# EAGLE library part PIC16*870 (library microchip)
MICROCONTROLLER flash type
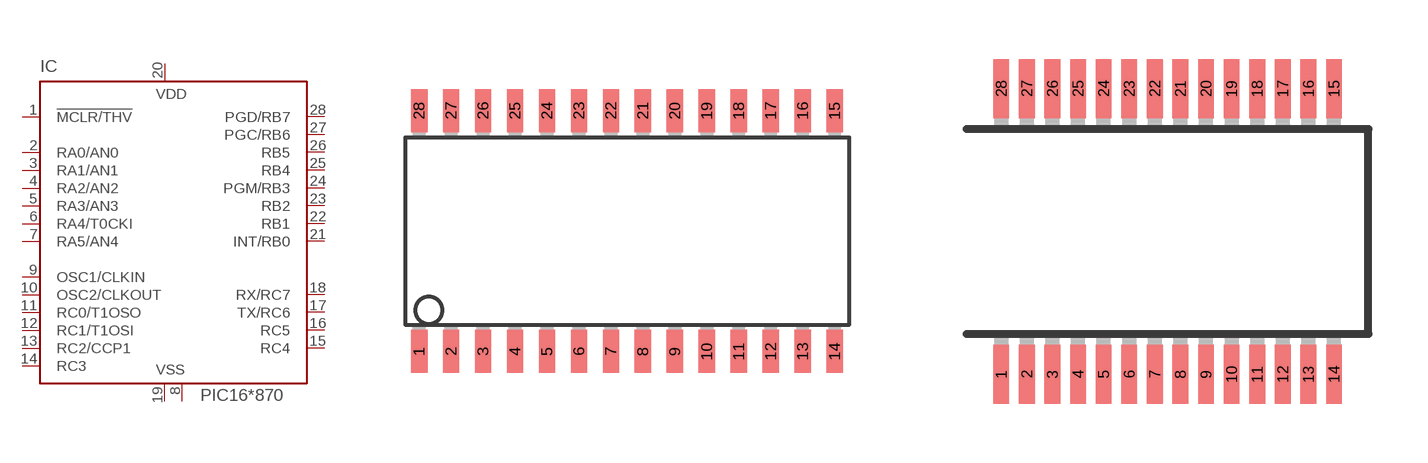
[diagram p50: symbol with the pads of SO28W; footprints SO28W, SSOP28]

Designator prefix IC

## PIC16F870SO (MF: MICROCHIP; MPN: PIC16F870-I/SO; OC_FARNELL: 9760946; OC_NEWARK: 61K3457), PIC16LF870SO (MF: MICROCHIP; MPN: PIC16LF870-I/SO; OC_FARNELL: 1815914; OC_NEWARK: 23C5702)  [SO28W]
1  !MCLR/THV  in
2  RA0/AN0
3  RA1/AN1
4  RA2/AN2
5  RA3/AN3
6  RA4/T0CKI
7  RA5/AN4
8  VSS  pwr
9  OSC1/CLKIN  in
10  OSC2/CLKOUT  out
11  RC0/T1OSO
12  RC1/T1OSI
13  RC2/CCP1
14  RC3
15  RC4
16  RC5
17  TX/RC6
18  RX/RC7
19  VSS  pwr
20  VDD  pwr
21  INT/RB0
22  RB1
23  RB2
24  PGM/RB3
25  RB4
26  RB5
27  PGC/RB6
28  PGD/RB7

## PIC16F870SS (MF: MICROCHIP; MPN: PIC16F870-I/SS; OC_FARNELL: 9760962; OC_NEWARK: 96K3885), PIC16LF870SS (MF: MICROCHIP; MPN: PIC16LF870-I/SS; OC_FARNELL: 1818506; OC_NEWARK: 23C5704)  [SSOP28]
Pads as for SO28W

## PIC16F870P (MF: MICROCHIP; MPN: PIC16F870-I/SP; OC_FARNELL: 9760954; OC_NEWARK: 19C7275), PIC16LF870P (MF: MICROCHIP; MPN: PIC16LF870-I/SP; OC_FARNELL: 1579594; OC_NEWARK: 69K7641)  [DIL28-3]
Pads as for SO28W

## Footprint SO28W (pad centres in mm)
28-Lead Plastic Small Outline (SO) Wide, 300 mil Body (SOIC) Source: http://ww1.microchip.com/downloads/en/devicedoc/39632c.pdf
smd 0.65 x 1.7: 1 -7.62,-4.78; 2 -6.35,-4.78; 3 -5.08,-4.78; 4 -3.81,-4.78; 5 -2.54,-4.78; 6 -1.27,-4.78; 7 0,-4.78; 8 1.27,-4.78; 9 2.54,-4.78; 10 3.81,-4.78; 11 5.08,-4.78; 12 6.35,-4.78; 13 7.62,-4.78; 14 8.89,-4.78; 15 8.89,4.78; 16 7.62,4.78; 17 6.35,4.78; 18 5.08,4.78; 19 3.81,4.78; 20 2.54,4.78; 21 1.27,4.78; 22 0,4.78; 23 -1.27,4.78; 24 -2.54,4.78; 25 -3.81,4.78; 26 -5.08,4.78; 27 -6.35,4.78; 28 -7.62,4.78

## Footprint SSOP28 (pad centres in mm)
Shrink Small Outline Package package type SS
smd 0.4 x 1.5: 1 -4.225,-3.625; 2 -3.575,-3.625; 3 -2.925,-3.625; 4 -2.275,-3.625; 5 -1.625,-3.625; 6 -0.975,-3.625; 7 -0.325,-3.625; 8 0.325,-3.625; 9 0.975,-3.625; 10 1.625,-3.625; 11 2.275,-3.625; 12 2.925,-3.625; 13 3.575,-3.625; 14 4.225,-3.625; 15 4.225,3.625; 16 3.575,3.625; 17 2.925,3.625; 18 2.275,3.625; 19 1.625,3.625; 20 0.975,3.625; 21 0.325,3.625; 22 -0.325,3.625; 23 -0.975,3.625; 24 -1.625,3.625; 25 -2.275,3.625; 26 -2.925,3.625; 27 -3.575,3.625; 28 -4.225,3.625

## Footprint DIL28-3 (pad centres in mm)
Dual In Line package type P
drill 0.813 long: 1 -16.51,-3.81; 2 -13.97,-3.81; 3 -11.43,-3.81; 4 -8.89,-3.81; 5 -6.35,-3.81; 6 -3.81,-3.81; 7 -1.27,-3.81; 8 1.27,-3.81; 9 3.81,-3.81; 10 6.35,-3.81; 11 8.89,-3.81; 12 11.43,-3.81; 13 13.97,-3.81; 14 16.51,-3.81; 15 16.51,3.81; 16 13.97,3.81; 17 11.43,3.81; 18 8.89,3.81; 19 6.35,3.81; 20 3.81,3.81; 21 1.27,3.81; 22 -1.27,3.81; 23 -3.81,3.81; 24 -6.35,3.81; 25 -8.89,3.81; 26 -11.43,3.81; 27 -13.97,3.81; 28 -16.51,3.81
